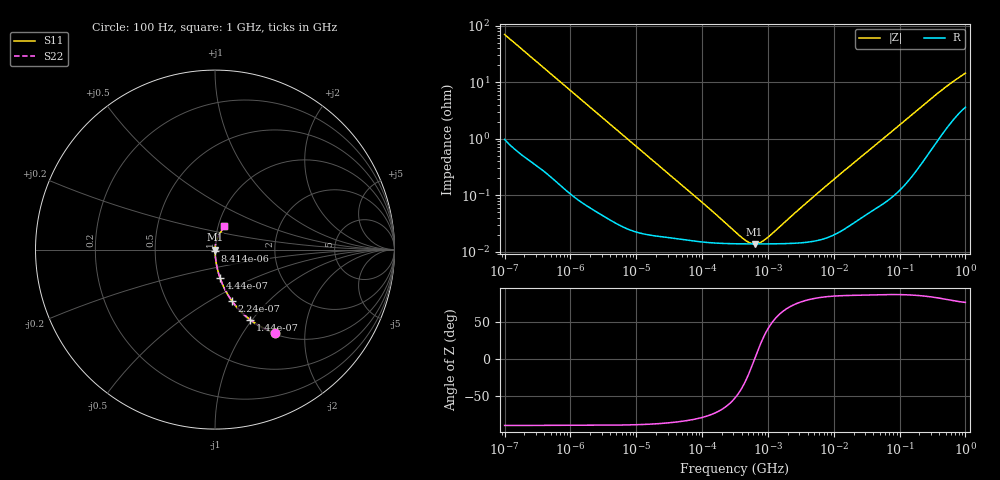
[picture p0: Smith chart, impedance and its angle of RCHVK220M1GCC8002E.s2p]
! RCHVK220M1GCC8002E  S-PARAMETER MODEL  (AEC-Q200 qualified)
! Model Generated by ELNA Corporation (http://www.ty-top.com)
! Version 1.0
! ELNA Control No. 201211
! Copyright (c) 2020 ELNA CO.,LTD. All Rights Reserved.
! Products Name : CONDUCTIVE POLYMER HYBRID ALUMINUM ELECTROLYTIC CAPACITORS
! Characteristics :
!  Capacitance  :  22uF  ,  Rated voltage  :  35V
!  Operating Temp. Range  :  -55 to +125 degC  ,  Endurance  :  4000hr at 125 degC
!  Dimension D  :  5mm  ,  Dimension L  :  5.8mm
! Frequency Range : 100Hz - 1GHz
! External Node Assignments :
!  1  o---| |---o  2
# MHz S RI R 50
!Freq[MHz].  S11 Real  S11 Imag  S21 Real  S21 Imag  S12 Real  S12 Imag  S22 Real  S22 Imag
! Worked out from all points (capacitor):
!   401 points, 100 Hz to 1 GHz, reference 50 ohm
!   read as one part in series: C = 22.6 uF near 108 Hz
!   lowest |Z| = 13.6 mohm at 627.3 kHz (marker M1)
!   series resonance near 629.1 kHz, so ESL is about 2.8 nH
!   S11 on the Smith chart (normalised r, x): 100 Hz: 1.02, -1.41; 144 Hz: 1.01, -0.98; 224 Hz: 1.01, -0.63; 444 Hz: 1.00, -0.32; 8.414 kHz: 1.00, -0.02; 1 GHz: 1.07, +0.28
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0.0001  0.3341 -0.4648  0.6659 0.4648  0.6659 0.4648  0.3341 -0.4648
0.000144  0.1974 -0.3916  0.8026 0.3916  0.8026 0.3916  0.1974 -0.3916
0.000224  0.094 -0.2851  0.906 0.2851  0.906 0.2851  0.094 -0.2851
0.000309  0.0529 -0.2167  0.9471 0.2167  0.9471 0.2167  0.0529 -0.2167
0.000444  0.0272 -0.1555  0.9728 0.1555  0.9728 0.1555  0.0272 -0.1555
0.000781  0.00963 -0.0906  0.9904 0.0906  0.9904 0.0906  0.00963 -0.0906
0.001488  0.00306 -0.0481  0.9969 0.0481  0.9969 0.0481  0.00306 -0.0481
0.008414  0.000311 -0.00865  0.9997 0.00865  0.9997 0.00865  0.000311 -0.00865
0.022131  0.000196 -0.0033  0.9998 0.0033  0.9998 0.0033  0.000196 -0.0033
0.115478  0.000146 -0.000628  0.9999 0.000628  0.9999 0.000628  0.000146 -0.000628
0.316228  0.000137 -0.000178  0.9999 0.000178  0.9999 0.000178  0.000137 -0.000178
0.473151  0.000136 -6.93e-05  0.9999 6.93e-05  0.9999 6.93e-05  0.000136 -6.93e-05
0.555904  0.000136 -2.98e-05  0.9999 2.98e-05  0.9999 2.98e-05  0.000136 -2.98e-05
0.627336  0.000136 -6.74e-07  0.9999 6.74e-07  0.9999 6.74e-07  0.000136 -6.74e-07
0.767361  0.000136 4.8e-05  0.9999 -4.8e-05  0.9999 -4.8e-05  0.000136 4.8e-05
0.977237  0.000136 0.000109  0.9999 -0.000109  0.9999 -0.000109  0.000136 0.000109
4.704354  0.000151 0.00088  0.9998 -0.00088  0.9998 -0.00088  0.000151 0.00088
69.9842  0.000991 0.0123  0.999 -0.0123  0.999 -0.0123  0.000991 0.0123
184.0772  0.00379 0.0316  0.9962 -0.0316  0.9962 -0.0316  0.00379 0.0316
395.8221  0.014 0.0641  0.986 -0.0641  0.986 -0.0641  0.014 0.0641
695.825  0.0334 0.1005  0.9666 -0.1005  0.9666 -0.1005  0.0334 0.1005
1000  0.0524 0.1287  0.9476 -0.1287  0.9476 -0.1287  0.0524 0.1287
